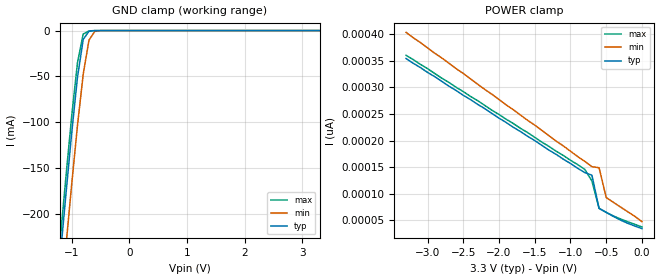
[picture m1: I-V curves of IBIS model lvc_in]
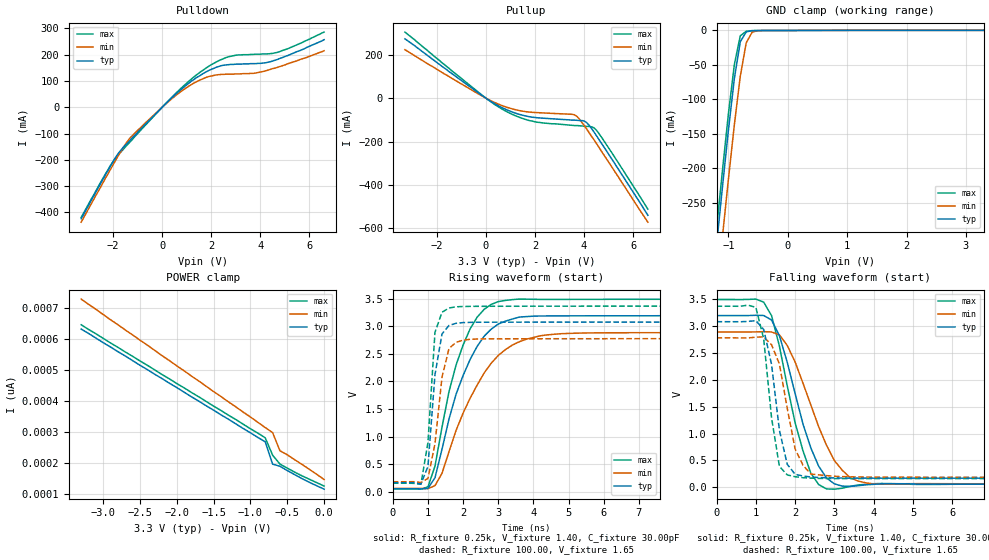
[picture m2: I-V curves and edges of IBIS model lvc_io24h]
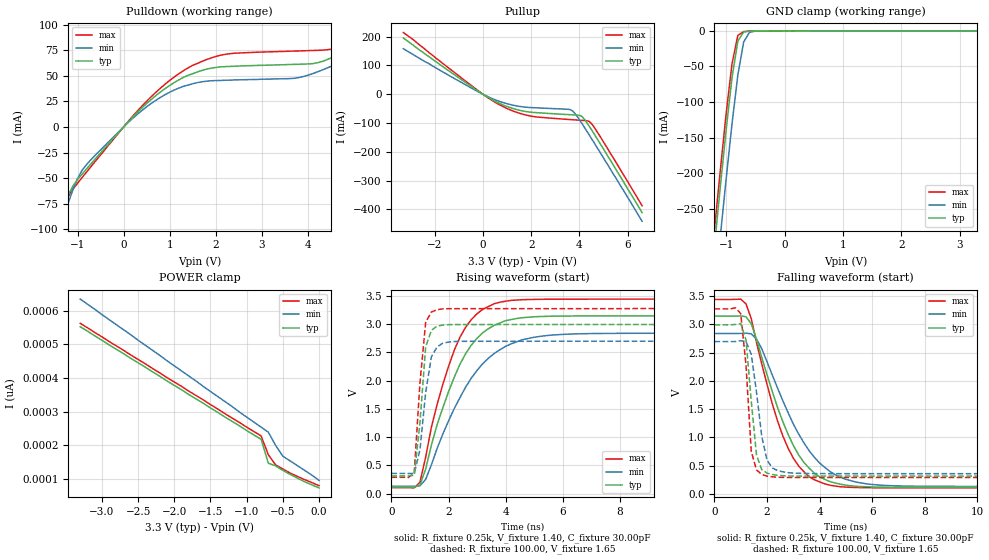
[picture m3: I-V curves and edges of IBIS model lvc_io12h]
| IBIS file 162245xh.ibs created by s2ibis2 version 1.1
| North Carolina State University Electronics Research Laboratory  1995
[IBIS ver]   2.1
[File name]   162245xh.ibs
[File Rev]   1.0
[Date]   03/01/99 rtk rtk
[Source]   Integrated Device Technology, Inc.
[Notes]   1.Temperatures: typ=25C, min=100C, max=0C 2.RRmp rates based
   on 50 ohm load.
[Disclaimer] Integrated Device Technology, Inc. ("IDT") hereby grants the
   user of this IBIS model a non-exclusive, nontransferable
   license to use this IBIS model under the following terms. The
   user is granted this license only to use the IBIS model and is
   not granted rights to sell, copy (except as needed to run the
   IBIS model), rent, lease or sub-license the IBIS model in
   whole or in part, or in modified form to anyone. The User may
   modify the IBIS model to suit its specific applications, but
   rights to derivative works and such modifications shall belong
   to IDT. This IBIS model is provided on an AS IS" basis and IDT
   makes absolutely no warranty with respect to the information
   contained herein. IDT DISCLAIMS AND CUSTOMER WAIVES ALL
   WARRANTIES, EXPRESS AND IMPLIED, INCLUDING WARRANTIES OF
   MERCHANTABILITY AND FITNESS FOR A PARTICULAR PURPOSE. THE
   ENTIRE RISK AS TO QUALITY AND PERFORMANCE IS WITH THE USER
   ACCORDINGLY, IN NO EVENT SHALL IDT BE LIABLE FOR ANY DIRECT OR
   INDIRECT DAMAGES, WHETHER IN CONTRACT OR TORT, INCLUDING ANY
   LOST PROFITS OR OTHER INCIDENTAL, CONSEQUENTIAL, EXEMPLARY, OR
   PUNITIVE DAMAGES ARISING OUT OF THE USE OR APPLICATION OF THE
   IBIS model. Further, IDT reserves the right to make changes
   without notice to any product herein to improve reliability,
   function, or design. IDT does not convey any license under
   patent rights or any other intellectual property rights,
   including those of third parties. IDT is not obligated to
   provide maintenance or support for the licensed IBIS model.
[Copyright]   Copyright 1997, Integrated Device Technology, Inc. all rights
   reserved
|   Component LVCH162245
[Component]   LVCH162245
[Manufacturer]   Integrated Device Technology
[Package]
| PA48
| variable   typ   min   max
R_pkg   6.50m   5.00m   10.00m
L_pkg   3.20nH   2.50nH   4.40nH
C_pkg   0.27pF   0.01pF   0.98pF
| PV48   typ   min   max
|R_pkg   6.5m   5.00m   10.00m
|L_pkg   4.75nH   3.82nH   6.72nH
|C_pkg   0.24pF   0.01pF   1.55pF
[Pin]  signal_name   model_name   R_pin   L_pin   C_pin
1   1DIR   lvc_in
2   1B1   lvc_io24h
3   1B2   lvc_io24h
4   GND   GND
5   1B3   lvc_io24h
6   1B4   lvc_io24h
7   VCC   POWER
8   1B5   lvc_io24h
9   1B6   lvc_io24h
10   GND   GND
11   1B7   lvc_io24h
12   1B8   lvc_io24h
13   2B1   lvc_io24h
14   2B2   lvc_io24h
15   GND   GND
16   2B3   lvc_io24h
17   2B4   lvc_io24h
18   VCC   POWER
19   2B5   lvc_io24h
20   2B6   lvc_io24h
21   GND   GND
22   2B7   lvc_io24h
23   2B8   lvc_io24h
24   2DIR   lvc_in
25   2OEB   lvc_in
26   2A8   lvc_io12h
27   2A7   lvc_io12h
28   GND   GND
29   2A6   lvc_io12h
30   2A5   lvc_io12h
31   VCC   POWER
32   2A4   lvc_io12h
33   2A3   lvc_io12h
34   GND   GND
35   2A2   lvc_io12h
36   2A1   lvc_io12h
37   1A8   lvc_io12h
38   1A7   lvc_io12h
39   GND   GND
40   1A6   lvc_io12h
41   1A5   lvc_io12h
42   VCC   POWER
43   1A4   lvc_io12h
44   1A3   lvc_io12h
45   GND   GND
46   1A2   lvc_io12h
47   1A1   lvc_io12h
48   1OEB   lvc_in
| Models and submodels in the file (3): lvc_in (Input), lvc_io24h (I/O), lvc_io12h (I/O)
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| in   in   dummy_model
| oe   oe
|   Model lvc_in
[Model]   lvc_in
Model_type   Input
Vinl =  0.800V
Vinh =  2.000V
C_comp   3.00pF   NA   NA
[Temperature Range]   25.00   100.00   0.000
[Voltage Range]   3.30V   3.00V   3.60V
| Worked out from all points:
|   GND clamp passes 1 mA (typ) near -0.70 V on its own axis
[GND_clamp]
| voltage   I(typ)   I(min)   I(max)
-3.3V     -1.806A    -1.858A    -1.789A
-1.2V     -248mA     -306mA     -229mA
-1.1V     -179mA     -236mA     -160mA
-1V       -112mA     -168mA     -93.56mA
-900mV    -51.39mA   -104mA     -35.36mA
-800mV    -9.697mA   -47.7mA    -3.786mA
-700mV    -714uA     -10.4mA    -348uA
-600mV    -52.42uA   -951uA     -8.225uA
-500mV    -126nA     -30.48uA   -10.89nA
3.3V      34.69pA    75.27pA    23pA
[POWER_clamp]
| voltage   I(typ)   I(min)   I(max)
-3.3V     354pA      403pA      360pA
-800mV    140pA      161pA      146pA
-700mV    135pA      151pA      124pA
-600mV    72.75pA    149pA      72.79pA
-500mV    65.09pA    93.05pA    65.39pA
-300mV    50.77pA    75.27pA    52.78pA
0V        34.68pA    47.91pA    37.83pA
|   Model lvc_io24h
[Model]   lvc_io24h
Model_type   I/O
Polarity   Non-Inverting
Enable   Active-High
Vinl =  0.000V
Vinh =  2.000V
Vmeas =  1.500V
C_comp   3.00pF   NA   NA
[Temperature Range]   25.00   100.00   0.000
[Voltage Range]   3.30V   3.00V   3.60V
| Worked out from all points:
|   slope of the pulldown table from 0 to 0.495 V, typ, clamps not added: 11.1 ohm
|   slope of the pullup table from 0 to 0.495 V, typ, clamps not added: 14.5 ohm
|   GND clamp passes 1 mA (typ) near -0.64 V on its own axis
|   rising waveform, R_fixture 0.25k, V_fixture 1.40, C_fixture 30.00pF: 20-80 % time 974ps typ, 1.24ns min, 819ps max; typ from 0.061 V to 3.19 V
|   rising waveform, R_fixture 100.00, V_fixture 1.65: 20-80 % time 266ps typ, 323ps min, 208ps max; typ from 0.171 V to 3.08 V
|   falling waveform, R_fixture 0.25k, V_fixture 1.40, C_fixture 30.00pF: 20-80 % time 725ps typ, 902ps min, 639ps max; typ from 3.19 V to 0.061 V
|   falling waveform, R_fixture 100.00, V_fixture 1.65: 20-80 % time 362ps typ, 397ps min, 304ps max; typ from 3.08 V to 0.171 V
[Pulldown]
| voltage   I(typ)   I(min)   I(max)
-3.3V     -424mA     -437mA     -419mA
-2.1V     -223mA     -235mA     -220mA
-1.8V     -177mA     -186mA     -182mA
-1.4V     -135mA     -128mA     -141mA
47.68nV   4.51nA     4.11nA     4.76nA
900mV     77.7mA     68.8mA     83.4mA
1.8V      135mA      114mA      150mA
2.6V      161mA      126mA      189mA
3.7V      166mA      129mA      201mA
4.4V      173mA      144mA      204mA
5.1V      196mA      165mA      222mA
6.6V      257mA      215mA      286mA
[Pullup]
| voltage   I(typ)   I(min)   I(max)
-3.3V     273mA      223mA      304mA
-200mV    15.7mA     12.6mA     17.8mA
800mV     -51.2mA    -39.9mA    -59.2mA
1.4V      -75.9mA    -58mA      -89.7mA
2V        -89.2mA    -66.1mA    -109mA
3.5V      -101mA     -74.3mA    -125mA
3.7V      -102mA     -83mA      -126mA
4.1V      -112mA     -141mA     -130mA
4.4V      -155mA     -191mA     -136mA
4.5V      -172mA     -208mA     -147mA
5.2V      -292mA     -329mA     -263mA
6.6V      -539mA     -571mA     -511mA
[GND_clamp]
| voltage   I(typ)   I(min)   I(max)
-3.3V     -2.217A    -2.283A    -2.195A
-1.2V     -312mA     -384mA     -288mA
-1.1V     -227mA     -299mA     -203mA
-1V       -145mA     -216mA     -121mA
-900mV    -69.9mA    -137mA     -49.49mA
-800mV    -16.48mA   -66.49mA   -7.75mA
-700mV    -2.021mA   -17.86mA   -1.171mA
-600mV    -313uA     -2.437mA   -215uA
-500mV    -136uA     -188uA     -155uA
3.3V      163uA      116uA      211uA
[POWER_clamp]
| voltage   I(typ)   I(min)   I(max)
-3.3V     631pA      728pA      645pA
-800mV    267pA      313pA      280pA
-700mV    195pA      297pA      224pA
-600mV    188pA      238pA      195pA
-300mV    148pA      194pA      157pA
0V        114pA      145pA      124pA
[Ramp]
| variable   typ   min   max
dV/dt_r   1.45/0.32n   1.21/0.34n   1.64/0.23n
dV/dt_f   1.59/0.39n   1.41/0.50n   1.76/0.35n
R_load = 50.00
[Rising Waveform]
R_fixture = 0.25k
V_fixture = 1.40
C_fixture = 30.00pF
R_dut = 7.00m
L_dut = 3.30nH
C_dut = 0.29pF
| time   V(typ)   V(min)   V(max)
0s        61.18mV    67.45mV    57.75mV
1ns       68.22mV    64.57mV    94.91mV
1.2ns     260mV      117mV      469mV
1.4ns     775mV      340mV      1.176V
1.6ns     1.324V     733mV      1.82V
2ns       2.108V     1.429V     2.659V
2.4ns     2.635V     1.936V     3.163V
3ns       3.038V     2.47V      3.444V
5ns       3.187V     2.869V     3.484V
19.8ns    3.189V     2.884V     3.487V
[Rising Waveform]
R_fixture = 100.00
V_fixture = 1.65
R_dut = 7.00m
L_dut = 3.30nH
C_dut = 0.29pF
| time   V(typ)   V(min)   V(max)
0s        171mV      188mV      161mV
800ps     147mV      174mV      143mV
1ns       463mV      248mV      895mV
1.2ns     2.124V     874mV      2.888V
1.4ns     2.86V      2.079V     3.252V
1.6ns     3.014V     2.598V     3.329V
1.8ns     3.052V     2.708V     3.35V
2ns       3.065V     2.747V     3.356V
2.6ns     3.071V     2.77V      3.359V
19.8ns    3.075V     2.775V     3.362V
[Falling Waveform]
R_fixture = 0.25k
V_fixture = 1.40
C_fixture = 30.00pF
R_dut = 7.00m
L_dut = 3.30nH
C_dut = 0.29pF
| time   V(typ)   V(min)   V(max)
0s        3.189V     2.884V     3.487V
1ns       3.194V     2.885V     3.495V
1.4ns     3.106V     2.884V     3.187V
1.8ns     2.32V      2.633V     1.883V
2.2ns     1.176V     1.933V     680mV
2.4ns     732mV      1.53V      262mV
2.8ns     175mV      780mV      -28.91mV
3.4ns     17.82mV    181mV      19.19mV
4ns       57.02mV    65.71mV    68.19mV
19.8ns    61.19mV    67.46mV    57.75mV
[Falling Waveform]
R_fixture = 100.00
V_fixture = 1.65
R_dut = 7.00m
L_dut = 3.30nH
C_dut = 0.29pF
| time   V(typ)   V(min)   V(max)
0s        3.075V     2.775V     3.362V
1ns       3.095V     2.788V     3.342V
1.2ns     2.931V     2.794V     2.759V
1.4ns     2.285V     2.647V     1.295V
1.6ns     1.061V     2.291V     390mV
1.8ns     428mV      1.467V     231mV
2ns       243mV      713mV      198mV
2.4ns     193mV      248mV      172mV
3.2ns     174mV      201mV      163mV
19.8ns    171mV      188mV      161mV
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|   Model lvc_io12h
[Model]   lvc_io12h
Model_type   I/O
Polarity   Non-Inverting
Enable   Active-High
Vinl =  0.000V
Vinh =  2.000V
Vmeas =  1.500V
C_comp   3.00pF   NA   NA
[Temperature Range]   25.00   100.00   0.000
[Voltage Range]   3.30V   3.00V   3.60V
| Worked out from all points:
|   slope of the pulldown table from 0 to 0.495 V, typ, clamps not added: 21.8 ohm
|   slope of the pullup table from 0 to 0.495 V, typ, clamps not added: 20.6 ohm
|   GND clamp passes 1 mA (typ) near -0.66 V on its own axis
|   rising waveform, R_fixture 0.25k, V_fixture 1.40, C_fixture 30.00pF: 20-80 % time 1.35ns typ, 1.68ns min, 1.16ns max; typ from 0.115 V to 3.15 V
|   rising waveform, R_fixture 100.00, V_fixture 1.65: 20-80 % time 266ps typ, 330ps min, 270ps max; typ from 0.313 V to 2.99 V
|   falling waveform, R_fixture 0.25k, V_fixture 1.40, C_fixture 30.00pF: 20-80 % time 1.44ns typ, 1.72ns min, 1.29ns max; typ from 3.15 V to 0.115 V
|   falling waveform, R_fixture 100.00, V_fixture 1.65: 20-80 % time 316ps typ, 418ps min, 270ps max; typ from 2.99 V to 0.313 V
[Pulldown]
| voltage   I(typ)   I(min)   I(max)
-3.3V     -374mA     -386mA     -370mA
-1.5V     -104mA     -116mA     -101mA
-1.4V     -90.3mA    -101mA     -88.3mA
-1.1V     -57.7mA    -61.4mA    -60.8mA
-600mV    -30.5mA    -26.9mA    -32.8mA
600mV     26.8mA     23mA       29.6mA
1.5V      52mA       42.2mA     60.2mA
2.3V      59.1mA     45.7mA     71.5mA
3.9V      61.4mA     49.2mA     74.4mA
4.6V      69.5mA     61mA       77mA
5.7V      96.7mA     84.7mA     104mA
6.6V      123mA      106mA      131mA
[Pullup]
| voltage   I(typ)   I(min)   I(max)
-3.3V     195mA      158mA      214mA
-300mV    16.6mA     13.3mA     18.8mA
700mV     -32.2mA    -25.2mA    -37.1mA
1.3V      -50.8mA    -38.9mA    -59.8mA
1.9V      -61.5mA    -45.8mA    -74.3mA
3.5V      -70.5mA    -52mA      -87.3mA
3.7V      -71.4mA    -56.7mA    -88.4mA
4.1V      -76.8mA    -101mA     -90.7mA
4.4V      -110mA     -140mA     -94mA
4.5V      -123mA     -154mA     -102mA
5.1V      -204mA     -235mA     -179mA
6.6V      -411mA     -441mA     -387mA
[GND_clamp]
| voltage   I(typ)   I(min)   I(max)
-3.3V     -2.169A    -2.233A    -2.148A
-1.2V     -303mA     -373mA     -279mA
-1.1V     -219mA     -289mA     -196mA
-1V       -139mA     -208mA     -116mA
-900mV    -65.88mA   -131mA     -46.16mA
-800mV    -14.28mA   -62.12mA   -6.236mA
-700mV    -1.456mA   -15.4mA    -849uA
-600mV    -262uA     -1.785mA   -208uA
-500mV    -136uA     -165uA     -155uA
3.3V      163uA      116uA      211uA
[POWER_clamp]
| voltage   I(typ)   I(min)   I(max)
-3.3V     552pA      634pA      562pA
-800mV    218pA      254pA      228pA
-700mV    147pA      239pA      172pA
-600mV    139pA      200pA      142pA
-500mV    126pA      168pA      130pA
-200mV    92.13pA    126pA      98.54pA
0V        73.94pA    96.21pA    80.65pA
[Ramp]
| variable   typ   min   max
dV/dt_r   1.26/0.25n   1.02/0.31n   1.46/0.27n
dV/dt_f   1.06/0.42n   0.85/0.53n   1.24/0.40n
R_load = 50.00
[Rising Waveform]
R_fixture = 0.25k
V_fixture = 1.40
C_fixture = 30.00pF
R_dut = 7.00m
L_dut = 3.30nH
C_dut = 0.29pF
| time   V(typ)   V(min)   V(max)
0s        115mV      132mV      106mV
1ns       150mV      140mV      201mV
1.2ns     435mV      252mV      645mV
1.6ns     1.217V     797mV      1.574V
2.2ns     2.056V     1.503V     2.535V
2.8ns     2.627V     2.044V     3.079V
3.6ns     2.976V     2.479V     3.359V
4.6ns     3.112V     2.724V     3.43V
6.2ns     3.141V     2.821V     3.439V
19.8ns    3.145V     2.838V     3.44V
[Rising Waveform]
R_fixture = 100.00
V_fixture = 1.65
R_dut = 7.00m
L_dut = 3.30nH
C_dut = 0.29pF
| time   V(typ)   V(min)   V(max)
0s        313mV      357mV      289mV
600ps     312mV      357mV      285mV
800ps     324mV      356mV      375mV
1ns       1.255V     776mV      1.959V
1.2ns     2.595V     1.787V     3.029V
1.4ns     2.887V     2.418V     3.213V
1.6ns     2.962V     2.595V     3.253V
1.8ns     2.981V     2.66V      3.267V
2.4ns     2.99V      2.693V     3.271V
19.8ns    2.991V     2.695V     3.273V
[Falling Waveform]
R_fixture = 0.25k
V_fixture = 1.40
C_fixture = 30.00pF
R_dut = 7.00m
L_dut = 3.30nH
C_dut = 0.29pF
| time   V(typ)   V(min)   V(max)
0s        3.145V     2.838V     3.44V
1.2ns     3.134V     2.844V     3.361V
1.4ns     3.011V     2.831V     3.101V
1.8ns     2.416V     2.568V     2.298V
2.4ns     1.529V     1.873V     1.291V
2.8ns     1.057V     1.439V     811mV
3.4ns     559mV      906mV      394mV
4.2ns     256mV      468mV      177mV
6.4ns     118mV      151mV      107mV
19.8ns    115mV      132mV      106mV
[Falling Waveform]
R_fixture = 100.00
V_fixture = 1.65
R_dut = 7.00m
L_dut = 3.30nH
C_dut = 0.29pF
| time   V(typ)   V(min)   V(max)
0s        2.991V     2.695V     3.273V
1ns       3.015V     2.709V     3.189V
1.2ns     2.722V     2.697V     2.275V
1.4ns     1.643V     2.471V     752mV
1.6ns     684mV      1.798V     424mV
1.8ns     428mV      1.014V     343mV
2ns       368mV      596mV      314mV
2.2ns     342mV      459mV      302mV
2.8ns     316mV      375mV      290mV
19.8ns    313mV      357mV      289mV
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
